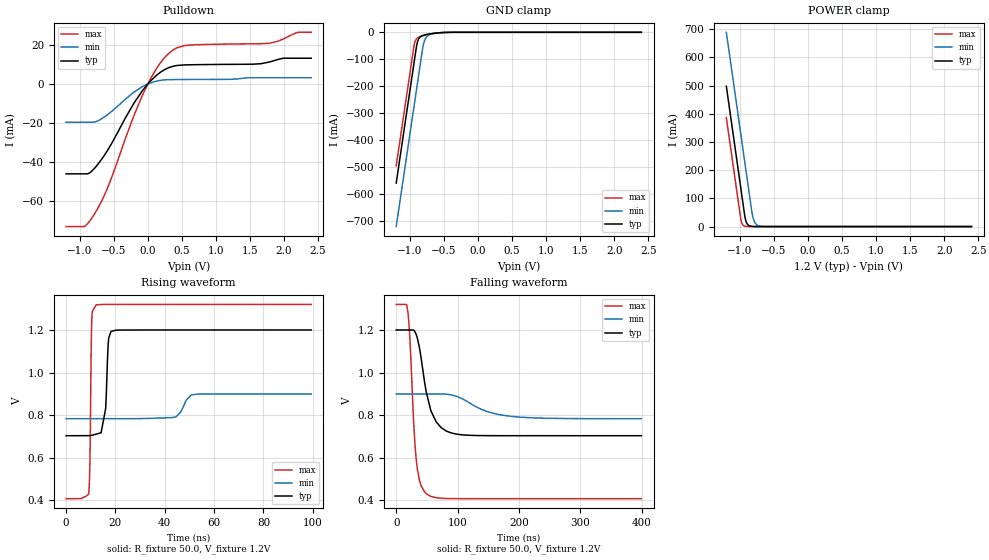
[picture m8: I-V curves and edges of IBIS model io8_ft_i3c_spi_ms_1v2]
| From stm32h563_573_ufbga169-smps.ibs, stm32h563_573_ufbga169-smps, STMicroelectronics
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[Model]   io8_ft_i3c_spi_ms_1v2
Model_type I/O_open_drain
Polarity   Non-Inverting
Enable   Active-Low
| CAP_THRESHOLD on pad IOFT is "UDTCAPC" :
| Rising=20.0% of vddiom   Falling=80.0% of vddiom
| C_comp min and max val. don't necessarily correlate with the min and max pvt
| but are the smallest and greatest pad capacitance found.
| var   typ   min   max
C_comp   3.41530pF  3.39695pF  3.42895pF
|C_comp_pulldown   3.41530pF  3.39695pF  3.42895pF
Vinl = 450.0mV
Vinh = 660.0mV
Vmeas = 600.0mV   | Reference voltage for timing measurements
Cref  = 50.0pF   | Timing specification test load capacitance value
Rref  = 1.0MOhm   | Timing specification test load resistance value
Vref  = 660.0mV   | Timing specification test load voltage
[Model Spec]
| TIME_THRESHOLD on pin ZII2CV11 is "CMOS" :
| Rising=40.0% of vdd   Falling=60.0% of vdd
Vinl 447.80000mV 344.80000mV 489.80000mV
Vinh 733.20000mV 535.20000mV 813.20000mV
| variable   typ   min   max
[Temperature Range] 25.0 125.0 -40.0
| variable   typ   min   max
[Voltage Range] 1.2V 900.0mV 1.32V
| variable   typ   min   max
[POWER Clamp Reference] 1.2V 900.0mV 1.32V
| variable   typ   min   max
[GND Clamp Reference] 0V 0V 0V
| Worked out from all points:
|   slope of the pulldown table from 0 to 0.18 V, typ, clamps not added: 30.6 ohm
|   GND clamp passes 1 mA (typ) near -0.52 V on its own axis
|   POWER clamp passes 1 mA (typ) near -0.84 V on its own axis
|   rising waveform, R_fixture 50.0, V_fixture 1.2V: 20-80 % time 1.34ns typ, 3.41ns min, 535ps max; typ from 0.704 V to 1.2 V
|   falling waveform, R_fixture 50.0, V_fixture 1.2V: 20-80 % time 20.7ns typ, 53.5ns min, 10ns max; typ from 1.2 V to 0.704 V
[POWER Clamp]
-1.2V     497.8mA    689.2mA    386.5mA
-990mV    140.8mA    332.2mA    29.53mA
-980mV    123.8mA    315.2mA    17.95mA
-960mV    89.81mA    281.2mA    6.634mA
-930mV    38.81mA    230.2mA    1.49mA
-900mV    12.07mA    179.2mA    334.8uA
-870mV    3.756mA    128.2mA    75.22uA
-820mV    536.4uA    44.98mA    6.246uA
-790mV    166.9uA    18.76mA    1.403uA
-750mV    35.18uA    5.846mA    191.8nA
-590mV    70.09nA    55uA       165.5pA
2.4V      0A         0A         0A
[GND Clamp]
-1.2V     -558.2mA   -719mA     -494.1mA
-940mV    -116.2mA   -277mA     -52.06mA
-930mV    -99.19mA   -260mA     -39.94mA
-900mV    -49.1mA    -209mA     -23.76mA
-880mV    -30.14mA   -175mA     -19.6mA
-850mV    -17.82mA   -124mA     -16.09mA
-810mV    -11.73mA   -56.78mA   -12.91mA
-780mV    -9.444mA   -28.21mA   -10.92mA
-740mV    -7.291mA   -13.16mA   -8.574mA
-640mV    -3.573mA   -4.171mA   -3.954mA
-380mV    -61.75uA   -230.3uA   -20.32uA
2.4V      3.863nA    718.4nA    150.6pA
| variable   typ   min   max
[Pullup Reference] 1.2V 900.0mV 1.32V
| variable   typ   min   max
[Pulldown Reference] 0V 0V 0V
[Pulldown]
-1.2V     -46.17mA   -19.62mA   -73.27mA
-930mV    -46.17mA   -19.62mA   -73.18mA
-770mV    -42.8mA    -19.41mA   -66.04mA
-570mV    -32.88mA   -15.18mA   -51.58mA
-200mV    -9.658mA   -4.083mA   -15.89mA
-80mV     -3.488mA   -1.363mA   -5.887mA
120mV     4.232mA    1.387mA    7.501mA
340mV     8.782mA    2.251mA    16.66mA
540mV     9.805mA    2.305mA    19.74mA
1.79V     11.33mA    3.206mA    20.93mA
2.2V      13.23mA    3.206mA    26.48mA
2.4V      13.23mA    3.206mA    26.56mA
[Ramp]
dV/dt_r 297.79736mV/1.03114ns 69.8957mV/3.06999ns 547.1337mV/533.04469ps
dV/dt_f 297.80514mV/20.20419ns 69.89965mV/53.11194ns 547.1393mV/10.02468ns
R_load = 50.0
| Removed startup time: 0s 0s 0s  .
| Removed end time: 99.4ns.
[Rising Waveform]
R_fixture   = 50.0
V_fixture   = 1.2V
V_fixture_min = 900.0mV
V_fixture_max = 1.32V
0s        703.7mV    783.5mV    408.1mV
9.1ns     704mV      783.5mV    428.2mV
9.65ns    704.4mV    783.5mV    570mV
10.15ns   705mV      783.5mV    1.083V
10.45ns   705.6mV    783.5mV    1.254V
12.2ns    711.1mV    783.5mV    1.318V
16.05ns   831.1mV    783.5mV    1.32V
17.1ns    1.136V     783.5mV    1.32V
18.25ns   1.194V     783.5mV    1.32V
99.4ns    1.2V       900mV      1.32V
| Removed startup time: 0s 0s 0s  .
| Removed end time: 399.4ns.
[Falling Waveform]
R_fixture   = 50.0
V_fixture   = 1.2V
V_fixture_min = 900.0mV
V_fixture_max = 1.32V
0s        1.2V       900mV      1.32V
18.75ns   1.2V       900mV      1.29V
21.8ns    1.2V       900mV      1.183V
32.6ns    1.178V     900mV      593.3mV
38.65ns   1.103V     900mV      486mV
48.9ns    909.4mV    900mV      431.9mV
65.2ns    768.5mV    900mV      412.5mV
97.8ns    711.4mV    889.2mV    408.3mV
187.5ns   703.7mV    794.6mV    408.1mV
399.4ns   703.7mV    783.5mV    408.1mV
